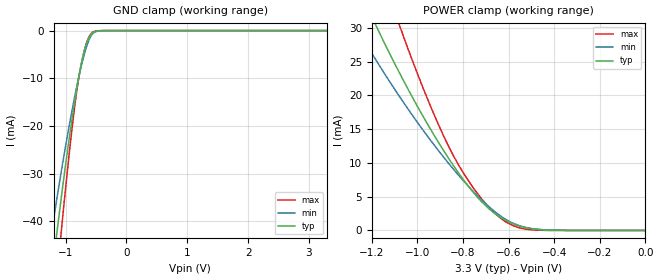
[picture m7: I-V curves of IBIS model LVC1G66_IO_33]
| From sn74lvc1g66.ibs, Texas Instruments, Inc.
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[Model]   LVC1G66_IO_33
Model_type  Terminator
| variable   typ   min   max
C_comp   4.50pF   0.35pF   6.54pF
| C_tri-state   4.50pF   0.35pF   6.54pF
[Temperature Range]   40   100   -40
| Ambient temperature   25   85   -40
[Voltage range]   3.3   3   3.6
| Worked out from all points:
|   GND clamp passes 1 mA (typ) near -0.59 V on its own axis
|   POWER clamp passes 1 mA (typ) near -0.58 V on its own axis
[GND Clamp]
| LVC1G66_IO_33
|   Voltage   I(typ)   I(min)   I(max)
-5.5V     -642.4mA   -532.1mA   -759.1mA
-1.23V    -51.42mA   -42.2mA    -63.45mA
-1.135V   -41.36mA   -34.43mA   -50.38mA
-1.075V   -35.27mA   -29.73mA   -42.41mA
-895mV    -18.49mA   -16.7mA    -20.48mA
-795mV    -10.5mA    -10.36mA   -10.76mA
-735mV    -6.458mA   -7.001mA   -6.532mA
-675mV    -3.355mA   -4.125mA   -3.355mA
-610mV    -1.339mA   -1.796mA   -1.168mA
-550mV    -454.4uA   -593.1uA   -293.5uA
-325mV    -1.323uA   -2.446uA   -114.8nA
3.3V      150.4pA    3.503uA    35.14pA
[POWER Clamp]
| LVC1G66_IO_33
|   Voltage   I(typ)   I(min)   I(max)
-5.5V     599.6mA    481.6mA    801mA
-1.265V   36.39mA    29.84mA    49.45mA
-1.175V   29.84mA    24.84mA    39.87mA
-1.085V   23.73mA    20.14mA    30.95mA
-1.055V   21.79mA    18.65mA    28.14mA
-940mV    14.84mA    13.24mA    18.18mA
-845mV    9.747mA    9.187mA    11.25mA
-740mV    5.038mA    5.242mA    5.607mA
-650mV    2.265mA    2.505mA    2.226mA
-580mV    972.3uA    1.063mA    700.8uA
-485mV    173.4uA    219uA      59.86uA
-95.1fV   150.4pA    905pA      41.76pA
